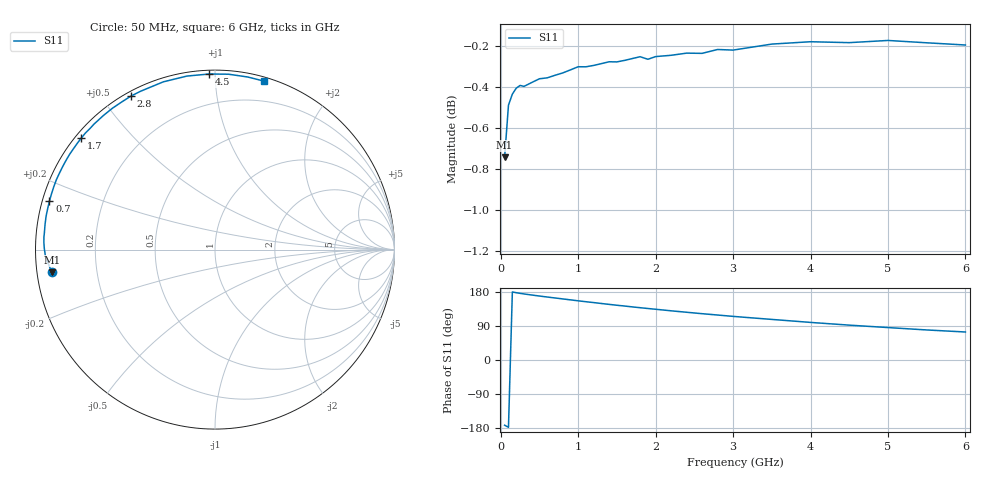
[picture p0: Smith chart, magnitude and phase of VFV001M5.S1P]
! Infineon Technologies  Discrete & RF Semiconductors
! BBY 58-03
! Si Tuning Diode in SOD323
! VR =
! S-Parameters:  June  1999
# GHz  S  MA  R  50
!  f  S11
! GHz  MAG  ANG
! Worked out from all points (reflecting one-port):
!   34 points, 50 MHz to 6 GHz, reference 50 ohm
!   lowest |S11| = -0.7 dB at 50 MHz (marker M1), VSWR 23.40, Z = 2.15 - j3.45 ohm
!   phase of S11 starts at -172 deg and turns -114 deg over the sweep
!   S11 on the Smith chart (normalised r, x): 50 MHz: 0.04, -0.07; 700 MHz: 0.02, +0.14; 1.7 GHz: 0.02, +0.36; 2.8 GHz: 0.02, +0.59; 4.5 GHz: 0.02, +0.97; 6 GHz: 0.03, +1.33
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0.05  0.918 -172.1
0.1  0.9452 -177.6
0.15  0.9511 179.6
0.2  0.9542 177.6
0.3  0.9552 174.3
0.4  0.9573 171.5
0.5  0.9593 168.8
0.7  0.9611 163.7
0.8  0.9624 161.2
1  0.9657 156.2
1.2  0.9665 151.5
1.3  0.9674 149.1
1.5  0.9684 144.5
1.6  0.9692 142.4
1.7  0.9702 140.1
1.8  0.9712 138.0
2  0.9712 133.9
2.2  0.972 129.8
2.4  0.9731 126.0
2.6  0.973 122.2
2.8  0.9751 118.7
3  0.9748 115.1
3.5  0.9781 107.1
4  0.9794 99.2
4.5  0.9789 92.0
5  0.9801 85.6
5.5  0.9788 79.3
6  0.9776 73.9
